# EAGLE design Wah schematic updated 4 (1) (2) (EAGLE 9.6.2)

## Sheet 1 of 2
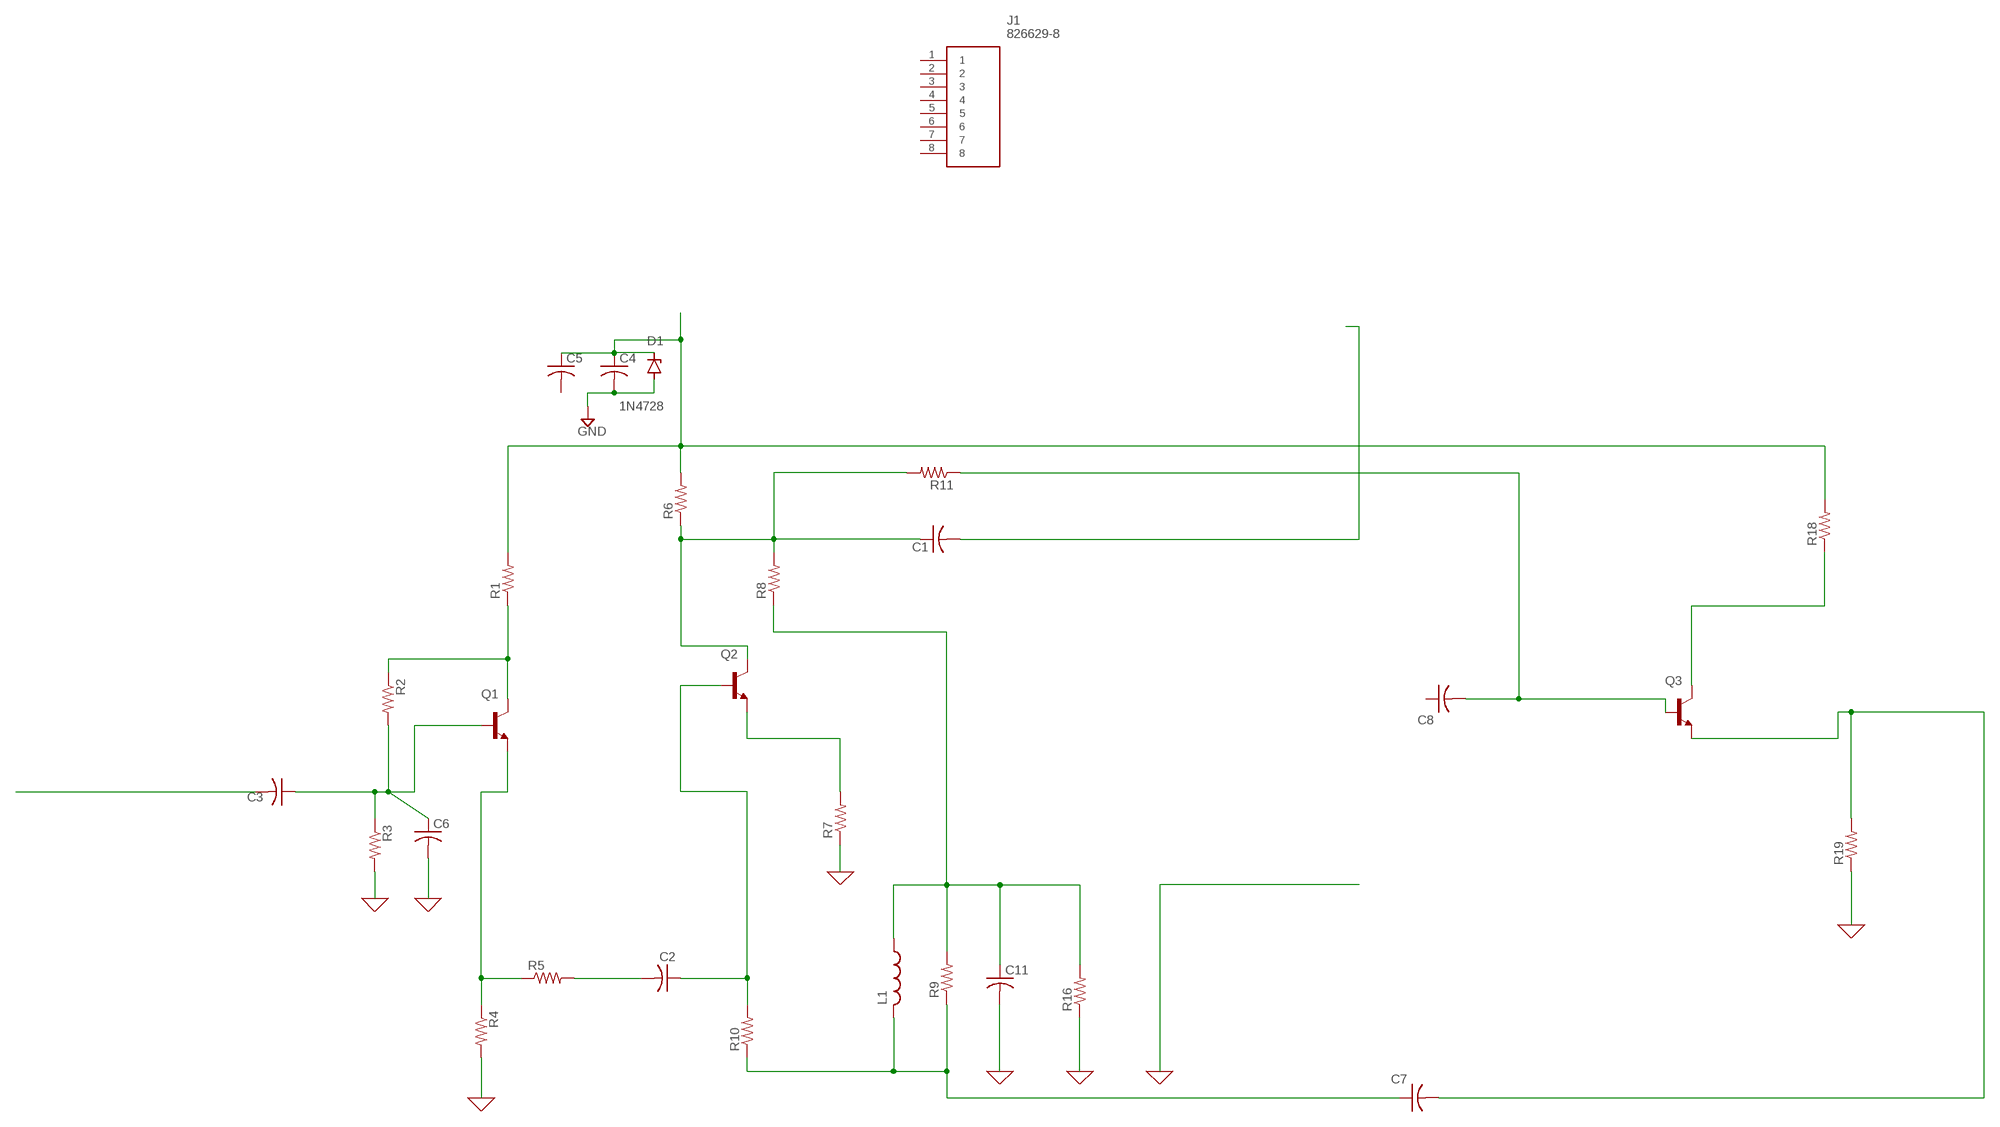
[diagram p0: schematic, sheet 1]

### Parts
C1  C-US050-024X044  [C050-024X044]
C2  C-US050-024X044  [C050-024X044]
C3  C-US050-024X044  [C050-024X044]
C4  C-US025-024X044  [C025-024X044]
C5  C-US025-024X044  [C025-024X044]
C6  C-US050-024X044  [C050-024X044]
C7  C-US050-024X044  [C050-024X044]
C8  C-US050-024X044  [C050-024X044]
C11  C-US050-024X044  [C050-024X044]
D1  1N4728  [DO41Z10]
J1  826629-8  [HDRV8W63P0X254_1X8_2032X250X95]
L1  L-US6000-XXX-RC  [6000-XXXX-RC]
Q1  -NPN-TO92  [TO92]
Q2  -NPN-TO92  [TO92]
Q3  -NPN-TO92  [TO92]
R1  R-US_0204/7  [0204/7]
R2  R-US_0204/7  [0204/7]
R3  R-US_0204/7  [0204/7]
R4  R-US_0204/7  [0204/7]
R5  R-US_0204/7  [0204/7]
R6  R-US_0204/7  [0204/7]
R7  R-US_0204/7  [0204/7]
R8  R-US_0204/7  [0204/7]
R9  R-US_0204/7  [0204/7]
R10  R-US_0204/7  [0204/7]
R11  R-US_0204/7  [0204/7]
R16  R-US_0204/7  [0204/7]
R18  R-US_0204/7  [0204/7]
R19  R-US_0204/7  [0204/7]

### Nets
0: C6.2 C11.2 R3.2 R4.2 R7.1 R16.1 R19.1 ; supply symbol labelled GND
GND: C4.2 D1.A
N$1: C3.1 C6.1 Q1.2(B) R2.2 R3.1
N$2: C1.1 Q2.3(C) R6.1 R8.2 R11.2
N$3: Q1.3(C) R1.1 R2.1
N$4: C7.1 L1.2 R9.1 R10.1
N$5: Q1.1(E) R4.1 R5.1
N$6: C2.1 Q2.2(B) R10.2
N$7: C1.2
N$8: Q2.1(E) R7.2
N$9: C11.1 L1.1 R8.1 R9.2 R16.2
N$12: C7.2 Q3.1(E) R19.2
N$13: C8.2 Q3.2(B) R11.1
N$14: C2.2 R5.2
N$15: C4.1 C5.1 D1.C R1.2 R6.2 R18.2
N$17: Q3.3(C) R18.1
N$18: C3.2
Unconnected: C5.2 C8.1 J1.1 J1.2 J1.3 J1.4 J1.5 J1.6 J1.7 J1.8

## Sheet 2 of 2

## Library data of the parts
C1-C8 C11 = rcl:C-US: CAPACITOR, American symbol; SPICEPREFIX: C
D1 = diode:1N4728: Z DIODE
J1 = SamacSys_Parts:826629-8: 8w Single row straight header gold Source: Datasheet; DESCRIPTION: 8w Single row straight header gold; HEIGHT: 9.5mm; MANUFACTURER_NAME: TE Connectivity; MANUFACTURER_PART_NUMBER: 826629-8; MOUSER_PART_NUMBER: 571-826629-8; MOUSER_PRICE-STOCK: https://www.mouser.co.uk/ProductDetail/TE-Connectivity/826629-8?qs=FazuUmncXokWopYWOwxkcA%3D%3D
L1 = rcl:L-US: INDUCTOR, American symbol; SPICEPREFIX: L
Q1-Q3 = transistor-neu-to92:*-NPN-: NPN Transistror
R1-R11 R16 R18 R19 = rcl:R-US_: RESISTOR, American symbol; SPICEPREFIX: R

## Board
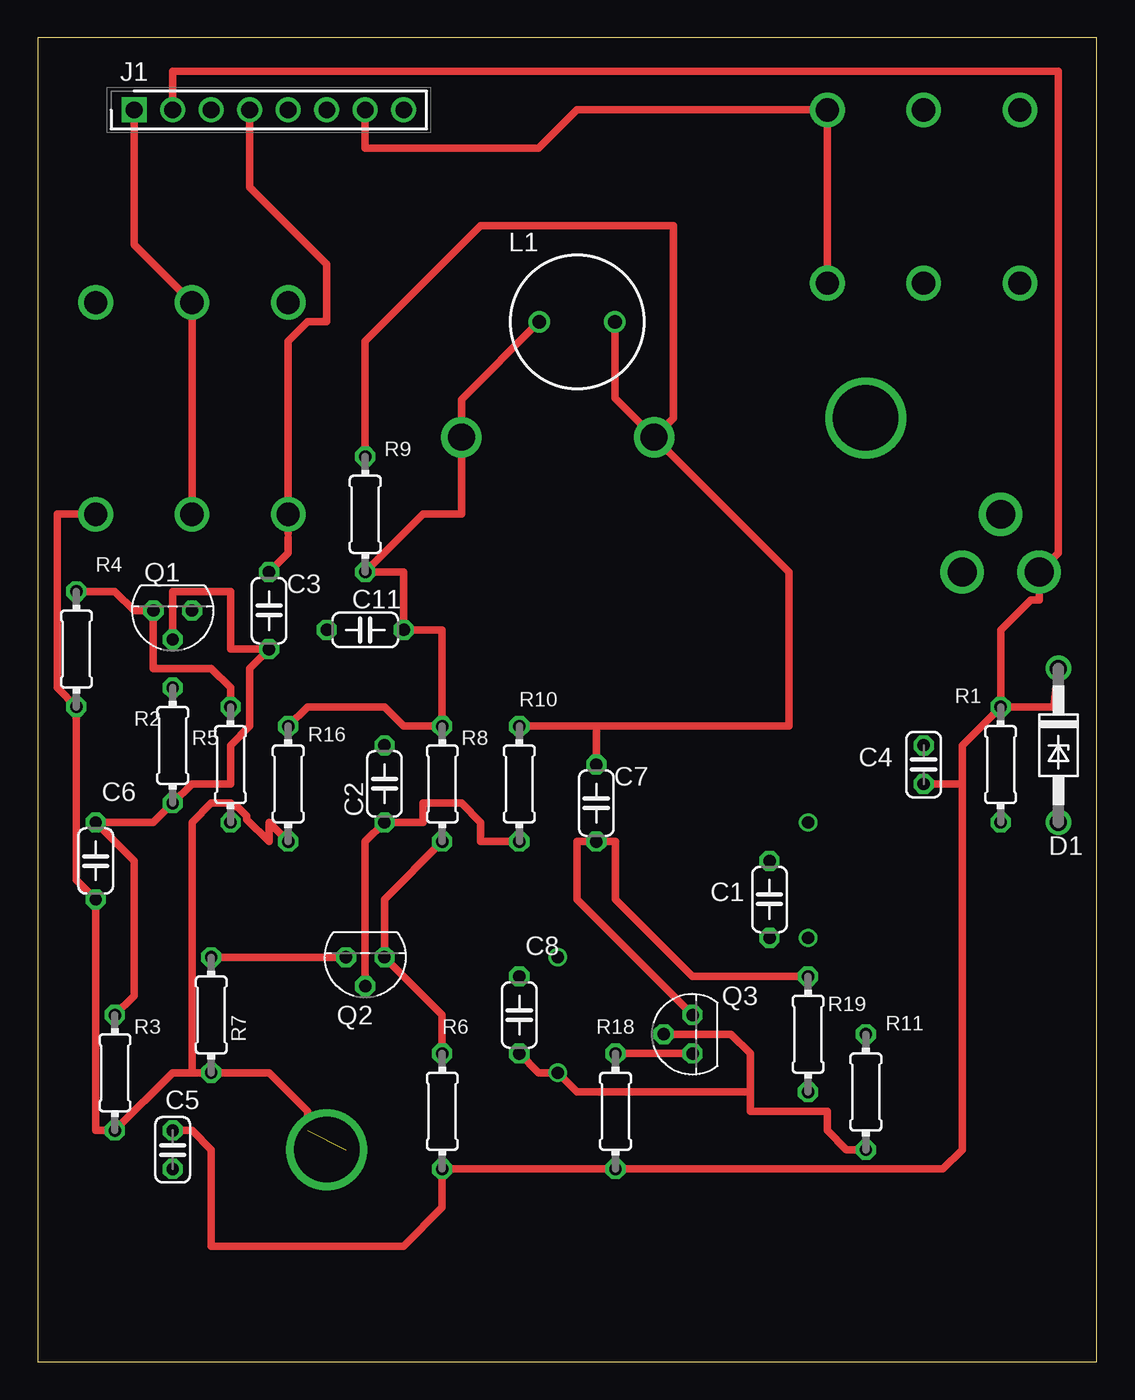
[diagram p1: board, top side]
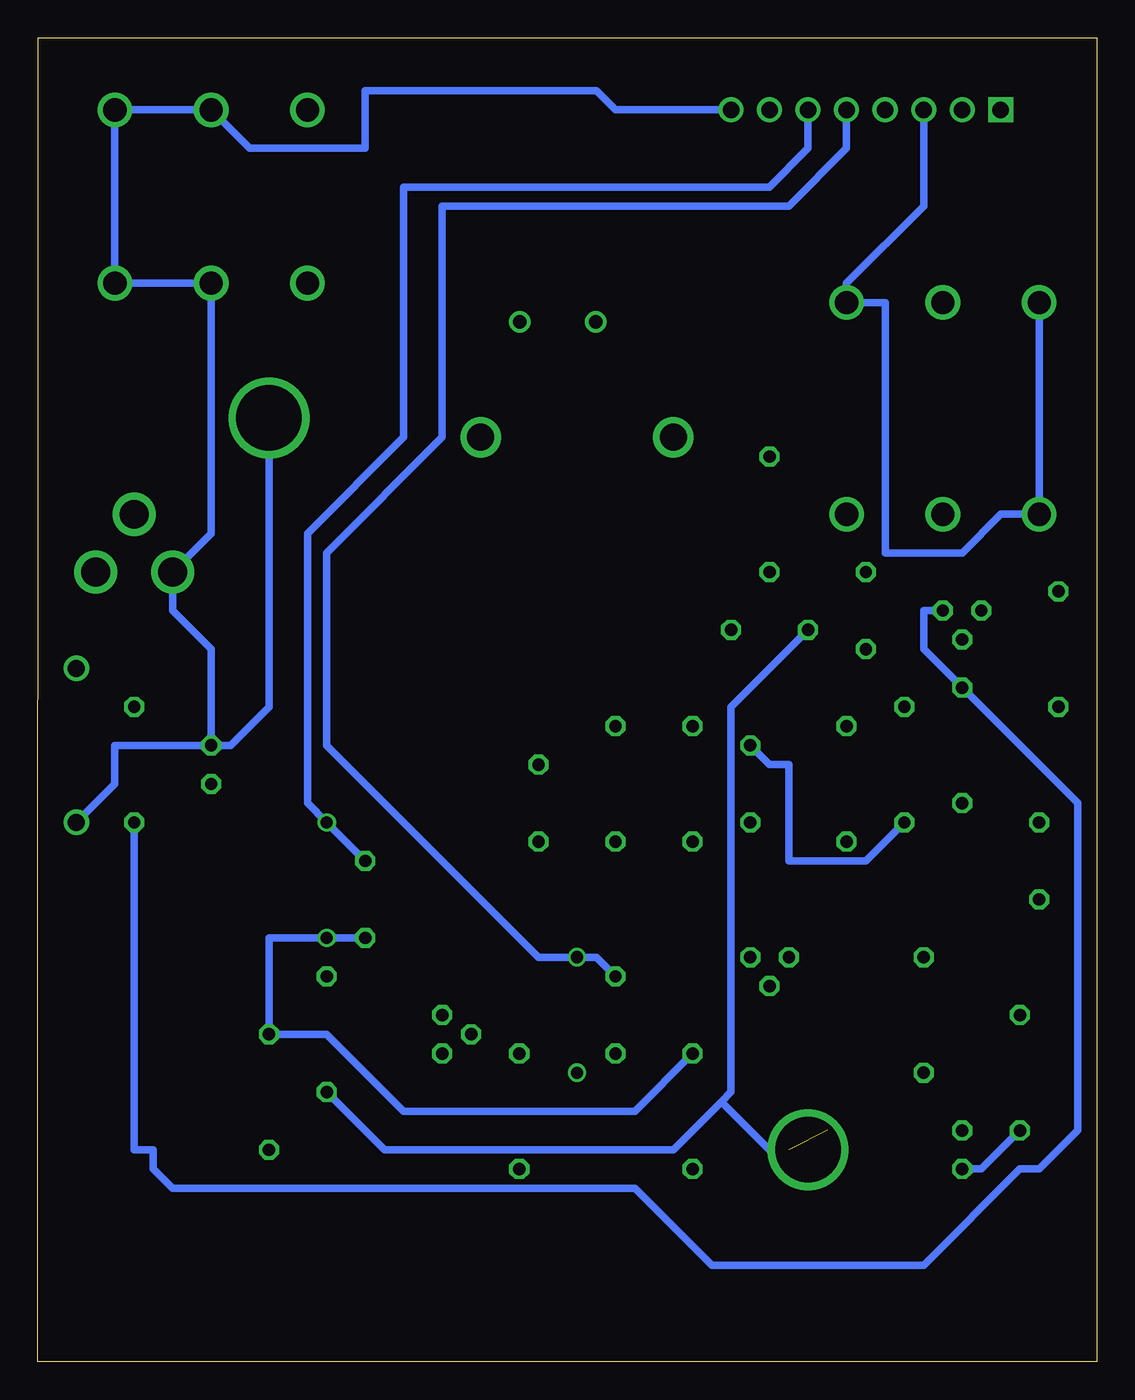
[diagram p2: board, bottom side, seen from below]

Size 69.85 x 87.3 mm. Coordinates in mm from the lower left corner, seen from the top.
Outline: 0,0 69.85,0 69.83,87.3 0,87.3 0,0
Copper layers (1*16): Top 0.035mm / dielectric 1.5mm / Bottom 0.035mm
Design rules "default": minimum track width 6mil, minimum drill 0.35mm, track to track 6mil, track to pad 6mil, pad to pad 6mil, via to via 6mil, smd to smd 6mil, copper to edge 40mil, drill to drill 6mil, minimum pad ring 10mil, minimum via ring 8mil, stop-mask expansion 4mil, vias tented up to drill 0mil, thermal gap 10mil

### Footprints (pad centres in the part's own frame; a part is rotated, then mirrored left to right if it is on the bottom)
C050-024X044 = drill 0.813 octagon: 1 -2.54,0; 2 2.54,0
C025-024X044 = drill 0.813 octagon: 1 -1.27,0; 2 1.27,0
DO41Z10 = drill 1.118: A 5.08,0; C -5.08,0
HDRV8W63P0X254_1X8_2032X250X95 = drill 1.1 pad 1.65 square: 1 0,0 | drill 1.1 pad 1.65: 2 2.54,0; 3 5.08,0; 4 7.62,0; 5 10.16,0; 6 12.7,0; 7 15.24,0; 8 17.78,0
6000-XXXX-RC = drill 0.9 pad 1.422: 1 -2.5,0; 2 2.5,0
TO92 = drill 0.813 octagon: 1 1.27,0; 2 0,1.905; 3 -1.27,0
0204/7 = drill 0.813 octagon: 1 -3.81,0; 2 3.81,0

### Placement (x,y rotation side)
C1  48.26,30.48 90 top
C2  22.86,38.1 90 top
C3  15.24,49.53 90 top
C4  58.42,39.37 90 top
C5  8.89,13.97 270 top
C6  3.81,33.02 270 top
C7  36.83,36.83 270 top
C8  31.75,22.86 270 top
C11  21.59,48.26 180 top
D1  67.31,40.64 270 top
J1  6.35,82.55 0 top
L1  35.56,68.58 0 top
Q1  8.89,49.53 180 top
Q2  21.59,26.67 180 top
Q3  43.18,21.59 90 top
R1  63.5,39.37 90 top
R2  8.89,40.64 270 top
R3  5.08,19.05 270 top
R4  2.54,46.99 270 top
R5  12.7,39.37 270 top
R6  26.67,16.51 270 top
R7  11.43,22.86 90 top
R8  26.67,38.1 270 top
R9  21.59,55.88 270 top
R10  31.75,38.1 270 top
R11  54.61,17.78 90 top
R16  16.51,38.1 90 top
R18  38.1,16.51 270 top
R19  50.8,21.59 90 top

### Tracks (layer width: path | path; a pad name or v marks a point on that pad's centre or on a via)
0  (1 unrouted)
  Top 0.508: 3.81,55.88 1.27,55.88 1.27,44.45 R4.2 2.54,31.75 C6.2 3.81,15.24 R3.2 8.89,19.05 10.16,19.05 | 10.16,19.05 R7.1 15.24,19.05 17.78,16.51 17.78,15.24 | 10.16,19.05 10.16,35.56 11.43,36.83 12.7,36.83 12.9,36.63 13.14,36.63 13.77,36 13.77,35.76 15.24,34.29 15.24,35.56 R16.1
  Bottom 0.508: C11.2 24.13,43.18 24.13,17.78 24.77,17.14 | 24.77,17.14 27.94,13.97 46.99,13.97 R19.1 | 24.77,17.14 21.59,13.97 20.32,13.97 | R3.2 7.62,12.7 8.89,12.7
GND
  Bottom 0.508: C4.2 64.77,40.64 64.77,38.1 D1.A | C4.2 57.15,40.64 54.61,43.18 54.61,60.96 | C4.2 58.42,46.99 60.96,49.53 60.96,52.07
N$1
  Top 0.508: R3.1 6.35,24.13 6.35,33.02 C6.1 7.62,35.56 R2.2 10.16,38.1 12.7,38.1 12.7,40.64 13.97,41.91 13.97,45.72 C3.1 12.7,46.99 12.7,50.8 8.89,50.8 Q1.2
N$2  (via drill 0.8)
  Top 0.508: R8.2 22.86,30.48 Q2.3 26.67,22.86 R6.1
  Bottom 0.508: R6.1 30.48,16.51 45.72,16.51 50.8,21.59 R11.2 54.61,27.94 v50.8,27.94 C1.1
N$3
  Bottom 0.508: R1.1 63.5,13.97 62.23,13.97 62.23,12.7 60.96,11.43 30.48,11.43 25.4,6.35 11.43,6.35 5.08,12.7 3.81,12.7 1.27,15.24 1.27,36.83 R2.1 11.43,46.99 11.43,49.53 Q1.3
N$4
  Top 0.508: R10.1 36.83,41.91 | 36.83,41.91 49.53,41.91 49.53,52.07 40.64,60.96 | L1.2 38.06,63.54 40.64,60.96 | R9.1 21.59,67.31 29.21,74.93 41.91,74.93 41.91,62.23 40.64,60.96 | 36.83,41.91 C7.1
N$5
  Top 0.508: R4.1 5.08,50.8 6.35,49.53 Q1.1 7.62,45.72 11.43,45.72 12.7,44.45 R5.1
N$6
  Top 0.508: Q2.2 21.59,34.29 C2.1 25.4,35.56 25.4,36.83 27.94,36.83 29.21,35.56 29.21,34.29 R10.2
N$8
  Top 0.508: R7.2 Q2.1
N$9
  Top 0.508: R16.2 17.78,43.18 22.86,43.18 24.13,41.91 R8.1 26.67,48.26 C11.1 24.13,52.07 R9.2 25.4,55.88 27.94,55.88 27.94,63.46 L1.1
N$10
  Bottom 0.508: 31.75,25.4 33.02,26.67 34.29,26.67
N$11  (via drill 1.78)
  other vias: 27.94,60.96
N$12
  Top 0.508: Q3.1 35.56,30.48 35.56,34.29 C7.2 38.1,34.29 38.1,30.48 43.18,25.4 R19.2
N$13  (via drill 0.8)
  Top 0.508: R11.1 53.34,13.97 52.07,15.24 52.07,16.51 46.99,16.51 46.99,17.78 | Q3.2 45.72,21.59 46.99,20.32 46.99,17.78 | C8.2 33.02,19.05 v34.29,19.05 35.56,17.78 46.99,17.78
N$14
  Bottom 0.508: R5.2 15.24,33.02 20.32,33.02 20.32,39.37 21.59,39.37 C2.2
N$15
  Top 0.508: 60.96,38.1 60.96,13.97 59.69,12.7 R18.2 R6.2 26.67,10.16 24.13,7.62 11.43,7.62 11.43,13.97 10.16,15.24 C5.1 | R1.2 60.96,40.64 60.96,38.1 | R1.2 63.5,48.26 65.47,50.23 66.04,50.23 66.04,52.07 | C4.1 60.96,38.1 | R1.2 66.99,43.18 D1.C
N$16  (via drill 1.52)
  Bottom 0.508: v3.81,55.88 6.35,55.88 8.89,53.34 13.97,53.34 13.97,69.85 16.51,69.85
N$17
  Top 0.508: R18.1 Q3.3
N$18
  Top 0.508: C3.2 16.51,53.34 16.51,54.33
N$19  (via drill 1.52)
  Bottom 0.508: v3.81,69.85 3.81,55.88
N$20  (via drill 1.52)
  Top 0.508: v10.16,55.88 10.16,69.85
N$21  (via drill 1.52)
  Bottom 0.508: v58.42,71.12 58.42,55.88
N$22  (via drill 1.52)
  Top 0.508: v10.16,69.85 6.35,73.66 6.35,82.55
N$23  (via drill 1.52)
  Bottom 0.508: v16.51,69.85 16.51,71.12 11.43,76.2 11.43,82.55
N$24  (via drill 1.52)
  Top 0.508: 16.51,54.61 v16.51,55.88 16.51,67.31 17.78,68.58 19.05,68.58 19.05,72.39 13.97,77.47 13.97,82.55
N$25
  Top 0.508: 8.89,82.55 8.89,85.09 67.31,85.09 67.31,53.34
N$26
  Top 0.508: 52.07,71.12 52.07,82.55 35.56,82.55 33.02,80.01 21.59,80.01 21.59,82.55
N$27  (via drill 1.52)
  other vias: 52.07,82.55
N$28  (via drill 1.52)
  Bottom 0.508: 59.69,71.12 64.77,71.12 64.77,82.55 v58.42,82.55 55.88,80.01 50.8,80.01
N$30  (via drill 1.91)
  other vias: 66.04,52.07
N$31  (via drill 1.52)
  other vias: 64.77,82.55
N$32  (via drill 0.8)
  Bottom 0.508: 16.51,82.55 16.51,80.01 20.32,76.2 43.18,76.2 43.18,60.96 50.8,53.34 50.8,40.64 36.83,26.67 v34.29,26.67
N$33  (via drill 0.8)
  Bottom 0.508: 48.26,33.02 v50.8,35.56 52.07,36.83 52.07,54.61 45.72,60.96 45.72,77.47 21.59,77.47 19.05,80.01 19.05,82.55
N$34  (via drill 1.52)
  other vias: 64.77,71.12
N$35
  Bottom 0.508: 24.13,82.55 31.75,82.55 33.02,83.82 48.26,83.82 48.26,80.01 50.8,80.01
N$36  (via drill 4.32)
  other vias: 54.61,62.23
N$37  (via drill 1.91)
  other vias: 63.5,55.88
N$38  (via drill 1.52)
  other vias: 52.07,71.12
N$40  (via drill 1.91)
  Bottom 0.508: 58.42,55.88 58.42,54.61 v60.96,52.07
N$41
  Top 0.508: 67.31,53.34 66.04,52.07
N$42  (via drill 1.78)
  other vias: 40.64,60.96
N$43  (via drill 4.32)
  other vias: 19.05,13.97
